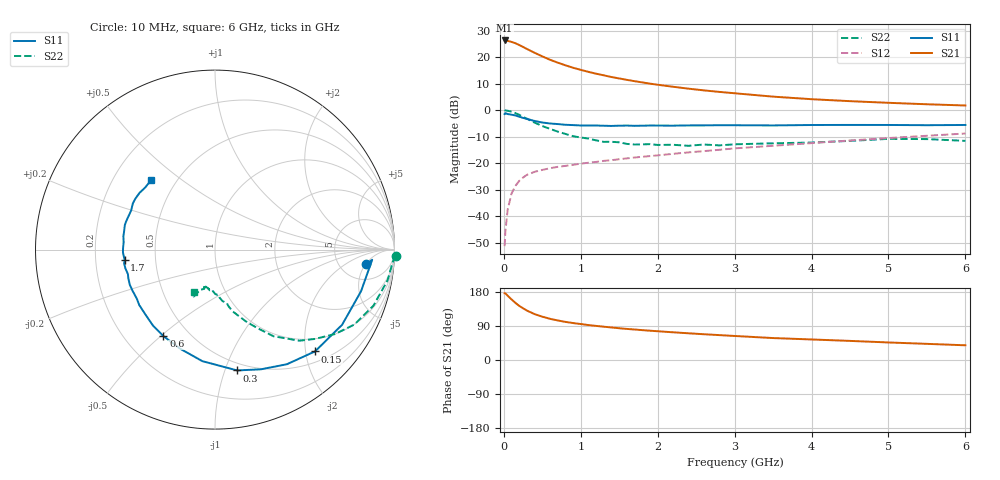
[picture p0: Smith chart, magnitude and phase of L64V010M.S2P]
!  INFINEON TECHNOLOGIES Small Signal Semiconductors
! BFR380L3 , Si-NPN RF-Transistor in TSLP-3-1
!  Vce=4 V,  Ic=10 mA
! Common Emitter S-Parameters:  07. March 2005
#  GHz  S  MA  R  50
! f  S11  S21  S12  S22
! GHz  Mag  Ang  Mag  Ang  Mag  Ang  Mag  Ang
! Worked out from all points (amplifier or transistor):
!   36 points, 10 MHz to 6 GHz, reference 50 ohm
!   highest |S21| = 26.3 dB at 10 MHz (marker M1)
!   |S21| within 3 dB of that: start of sweep to 286 MHz
!   unconditionally stable (mu >= 1): 2.322 GHz to 4.704 GHz
!   at 250 MHz: K = 0.24, MSG = 24.7 dB, |S12| = -25.4 dB
!   at 1.4 GHz: K = 0.85, MSG = 15.7 dB, |S12| = -18.9 dB
!   at 6 GHz: K = 0.96, MSG = 5.3 dB, |S12| = -8.8 dB
!   S11 on the Smith chart (normalised r, x): 10 MHz: 9, -5; 150 MHz: 0.71, -2.19; 300 MHz: 0.44, -1.10; 600 MHz: 0.36, -0.51; 1.7 GHz: 0.33, -0.05; 6 GHz: 0.36, +0.39
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0.01  0.8449 -5.6  20.76 176.0  0.0027 85.4  1.007 -2.0
0.02  0.8776 -3.7  20.68 175.9  0.0051 84.1  0.992 -4.1
0.05  0.8462 -15.9  20.38 169.6  0.0133 83.7  0.977 -10.0
0.1  0.8228 -30.6  19.5 159.9  0.0266 74.6  0.9364 -19.5
0.15  0.7952 -45.5  18.41 150.8  0.0372 68.2  0.8814 -28.3
0.2  0.7539 -57.9  17.02 142.9  0.0462 63.3  0.8177 -35.1
0.25  0.7144 -69.0  15.68 136.4  0.0535 58.6  0.7478 -41.7
0.3  0.6845 -79.6  14.34 130.4  0.0601 55.2  0.6918 -47.2
0.4  0.6254 -96.5  12.15 121.1  0.0685 51.2  0.5824 -56.0
0.5  0.5851 -109.5  10.38 114.3  0.0745 48.6  0.5023 -61.2
0.6  0.5611 -120.8  8.97 108.7  0.0801 47.3  0.4434 -66.1
0.7  0.5468 -129.1  7.912 104.4  0.085 47.2  0.3943 -70.2
0.8  0.5306 -136.7  7.05 100.6  0.0887 47.2  0.3565 -74.2
1.1  0.5134 -153.0  5.295 92.2  0.1018 49.0  0.291 -81.5
1.4  0.5041 -164.3  4.233 85.9  0.1137 51.1  0.253 -86.8
1.7  0.5065 -173.5  3.53 80.5  0.1276 53.4  0.2247 -93.5
2.2  0.5106 175.4  2.772 73.1  0.1499 55.8  0.2221 -98.8
2.8  0.5206 164.8  2.217 65.7  0.1787 58.6  0.2163 -106.4
3.5  0.5155 155.0  1.803 57.9  0.2128 59.1  0.237 -109.5
4.5  0.5268 147.3  1.481 50.4  0.2678 60.4  0.2634 -112.6
5.5  0.5206 138.3  1.294 42.6  0.3289 58.8  0.2844 -115.0
6  0.5259 132.6  1.227 38.8  0.3626 57.4  0.2635 -116.5
